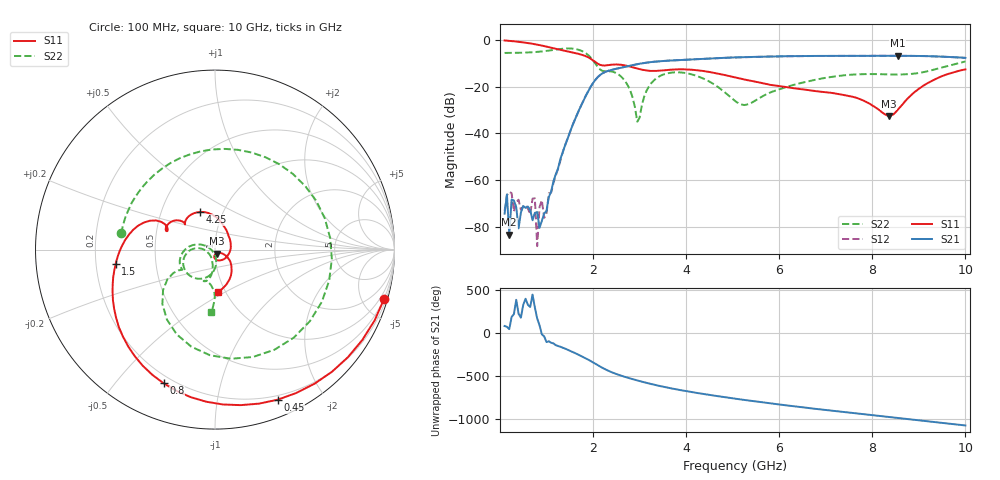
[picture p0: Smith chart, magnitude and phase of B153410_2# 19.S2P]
!  2-Port S-parameters saved by WinCal
! VAR MeasName=S-Parameters (CALIBRATED_DATA) read from VNA (N5245A)
! VAR MeasDate=2016-12-23 10:00:18
! VAR NAME=B153410_2# 19
! VAR FILENAME=B153410_2# 19.S2P
! VAR DATE=2016-12-23 10:00:18
! VAR PHYS_PORTS=1,2
# Hz S DB R 50
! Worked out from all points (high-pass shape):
!   199 points, 100 MHz to 10 GHz, reference 50 ohm
!   highest |S21| = -6.73 dB at 8.55 GHz (marker M1); lowest = -83.5 dB at 200 MHz (marker M2)
!   |S21| within 3 dB of the highest: 3.127 GHz to end of sweep
!   lowest |S11| = -32.5 dB at 8.35 GHz (marker M3), VSWR 1.05, Z = 50.9 - j2.23 ohm
!   |S11| at or under -10 dB: 2.092 GHz to end of sweep
!   |S22| runs from -35.0 to -3.6 dB; largest |S21 - S12| = 0.0027
!   S11 on the Smith chart (normalised r, x): 100 MHz: 0.47, -7.01; 450 MHz: 0.16, -1.49; 800 MHz: 0.16, -0.67; 1.5 GHz: 0.28, -0.06; 4.25 GHz: 0.78, +0.35; 10 GHz: 0.92, -0.46
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1e8  -0.16 -16.2  -74.44 85.8  -73.26 -21.2  -5.51 170.2
1.5e8  -0.24 -23.9  -66.22 76.3  -66.62 19.3  -5.51 165.3
2e8  -0.33 -31.5  -83.52 49.6  -65.11 100.5  -5.50 160.3
2.5e8  -0.42 -39.0  -68.44 -169.7  -65.63 87.8  -5.51 155.3
3e8  -0.52 -46.3  -68.80 -134.7  -73.50 -147.5  -5.48 150.3
4e8  -0.74 -60.5  -80.80 -131.3  -68.49 -1.4  -5.45 139.8
4.5e8  -0.85 -67.3  -74.02 -176.5  -72.83 37.3  -5.43 134.4
7.5e8  -1.77 -105.3  -74.12 -57.4  -67.85 15.7  -5.14 98.3
8e8  -1.96 -111.0  -73.77 173.8  -88.41 -45.7  -5.06 91.5
9e8  -2.36 -121.9  -77.58 -10.9  -68.73 -100.6  -4.88 77.1
1e9  -2.80 -131.9  -73.25 -101.4  -74.61 -79.7  -4.64 61.4
1.5e9  -5.05 -172.0  -39.66 158.3  -39.83 159.7  -3.58 -37.0
1.75e9  -6.25 170.2  -27.85 95.2  -27.80 95.2  -4.60 -92.8
2.65e9  -10.73 148.0  -11.63 -140.7  -11.62 -140.8  -16.62 173.9
2.95e9  -12.22 139.6  -10.33 171.8  -10.34 171.6  -35.02 -168.4
3.4e9  -13.16 139.5  -9.14 111.1  -9.13 111.1  -15.86 -106.7
4.25e9  -12.97 111.3  -8.16 24.7  -8.18 24.6  -15.57 -169.8
5.05e9  -16.00 78.4  -7.43 -40.6  -7.46 -40.5  -26.10 -170.7
6.7e9  -21.65 -10.6  -6.81 -154.1  -6.82 -154.0  -17.36 -97.6
8.35e9  -32.51 -67.7  -6.77 106.2  -6.76 106.4  -14.71 -108.7
8.55e9  -29.85 -35.2  -6.73 94.4  -6.74 94.4  -14.79 -106.7
1e10  -12.57 -86.2  -7.64 7.2  -7.62 7.4  -9.20 -93.7
